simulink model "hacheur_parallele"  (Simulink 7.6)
settings: Solver=ode15s  StartTime=0.0  StopTime=20  RelTol=1e-3
InitFcn:
  | clc
StopFcn:
  | clc
  | close all, clc
  | load U_Umoy_charge.mat
  | plot(x(1,:),x(2,:),x(1,:),x(3,:))
  | xlabel('temps')
  | title('Tension charge et sa valeur moyenne')
  | grid
  | 
  | load I_Imoy_charge.mat
  | figure
  | plot(y(1,:),y(2,:),y(1,:),y(3,:))
  | xlabel('temps')
  | title('Courant charge et sa valeur moyenne')
  | grid
  | 
  | delete *.mat
libraries: fl_lib x15, powerlib x13, nesl_utility x6, elec_lib x4, powerlib_extras x2

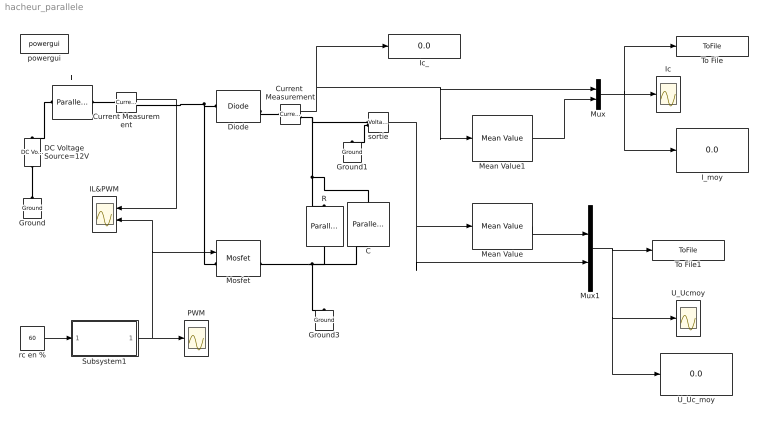
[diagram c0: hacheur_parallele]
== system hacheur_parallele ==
  C : powerlib/Elements/Parallel RLC Branch  DialogController=POWERSYS.PowerSysDialog  PhysicalDomain=powersysdomain  SubClassName=unknown  LeftPortType=p1  RightPortType=p1  LConnTagsString=a  RConnTagsString=__new0  BranchType=C  Resistance=1  Inductance=1e-3  SetiL0=off  InitialCurrent=0  Capacitance=100e-3  Setx0=off  InitialVoltage=0  Measurements=None
  Current Measurement : powerlib/Measurements/Current Measurement  DialogController=POWERSYS.PowerSysDialog  SystemSampleTime=-1  PhasorSimulation=off  OutputType=Complex  PSBequivalent=0
  Current  Measurement : powerlib/Measurements/Current Measurement  DialogController=POWERSYS.PowerSysDialog  SystemSampleTime=-1  PhasorSimulation=off  OutputType=Complex  PSBequivalent=0
  DC Voltage  Source=12V : powerlib/Electrical Sources/DC Voltage Source  DialogController=POWERSYS.PowerSysDialog  SystemSampleTime=-1  Amplitude=12  Measurements=None
  Diode : powerlib/Power Electronics/Diode  DialogController=POWERSYS.PowerSysDialog  SystemSampleTime=-1  Ron=0.001  Lon=0  Vf=0.8  IC=0  UseSnubber=off  Rs=500  Cs=250e-9  Measurements=on
  Ground : powerlib/Elements/Ground  DialogController=POWERSYS.PowerSysDialog  PhysicalDomain=powersysdomain  SubClassName=unknown  LeftPortType=p1  RightPortType=p1  LConnTagsString=a
  Ground1 : powerlib/Elements/Ground  DialogController=POWERSYS.PowerSysDialog  PhysicalDomain=powersysdomain  SubClassName=unknown  LeftPortType=p1  RightPortType=p1  LConnTagsString=a
  Ground3 : powerlib/Elements/Ground  DialogController=POWERSYS.PowerSysDialog  PhysicalDomain=powersysdomain  SubClassName=unknown  LeftPortType=p1  RightPortType=p1  LConnTagsString=a
  IL&PWM : Scope  NumInputPorts=2
  I_moy : Display
  Ic : Scope
  Ic_ : Display
  L : powerlib/Elements/Parallel RLC Branch  DialogController=POWERSYS.PowerSysDialog  PhysicalDomain=powersysdomain  SubClassName=unknown  LeftPortType=p1  RightPortType=p1  LConnTagsString=a  RConnTagsString=__new0  BranchType=L  Resistance=50  Inductance=1  SetiL0=off  InitialCurrent=0  Capacitance=25e-06  Setx0=off  InitialVoltage=0  Measurements=Branch voltage and current
  Mean Value : powerlib_extras/Measurements/Mean Value  DialogController=POWERSYS.PowerSysDialog  SystemSampleTime=-1  Period=10
  Mean Value1 : powerlib_extras/Measurements/Mean Value  DialogController=POWERSYS.PowerSysDialog  SystemSampleTime=-1  Period=10
  Mosfet : powerlib/Power Electronics/Mosfet  DialogController=POWERSYS.PowerSysDialog  SystemSampleTime=-1  Ron=0.1  Lon=0  Rd=0.01  Vfd=0  IC=0  Rs=1e5  Cs=inf  Measurements=on
  Mux : Mux  Inputs=2
  Mux1 : Mux  Inputs=2
  PWM : Scope
  R : powerlib/Elements/Parallel RLC Branch  DialogController=POWERSYS.PowerSysDialog  PhysicalDomain=powersysdomain  SubClassName=unknown  LeftPortType=p1  RightPortType=p1  LConnTagsString=a  RConnTagsString=__new0  BranchType=R  Resistance=10  Inductance=1.0  SetiL0=off  InitialCurrent=0  Capacitance=25e-06  Setx0=off  InitialVoltage=0  Measurements=Branch voltage and current
  Subsystem1 : Subsystem
  To File : ToFile  Filename=I_Imoy_charge  MatrixName=y
  To File1 : ToFile  Filename=U_Umoy_charge  MatrixName=x
  U_Uc_moy : Display
  U_Ucmoy : Scope
  powergui : powerlib/powergui  SystemSampleTime=-1  SimulationMode=Continuous  SampleTime=0  frequency=60  SPID=off  DisableSnubberDevices=off  DisableRonSwitches=off  DisableVfSwitches=off  SwTol=0  Interpol=off  frequencyindice=0  echomessages=off  HookPort=off  DisplayEquations=off  FunctionMessages=off  EnableUseOfTLC=off  x0status=blocks  RestoreLinks=warning  ResistiveCurrentMeasurement=off  Frange=[0:2:500]  Ylog=off  Xlog=on  ShowGrid=off  save=off  variable=ZData  ZoomFFT=on  StartTime=0.0  cycles=1  DisplayStyle=1  fundamental=60  FreqAxis=off  MaxFrequency=1000  frequencyindicesteady=1  RmsSteady=1  display=off  Ts=0  methode=off
  rc en % : Constant  Value=60
  sortie : powerlib/Measurements/Voltage Measurement  DialogController=POWERSYS.PowerSysDialog  SystemSampleTime=-1  PhasorSimulation=off  OutputType=Complex  PSBequivalent=0
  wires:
  rc en %/1 -> Subsystem1/1(rc (%))
  sortie/1 -> Mean Value/1, Mux1/2
  Current  Measurement/1 -> Ic_/1, Mean Value1/1, Mux/1
  Mean Value1/1 -> Mux/2
  Mux/1 -> Ic/1, To File/1, I_moy/1
  Subsystem1/1(PWM) -> PWM/1, Mosfet/1, IL&PWM/2
  Mean Value/1 -> Mux1/1
  Mux1/1 -> To File1/1, U_Uc_moy/1, U_Ucmoy/1
  Current Measurement/1 -> IL&PWM/1
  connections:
  DC Voltage  Source=12V/LConn1 -- Ground/LConn1
  Mosfet/RConn1 -- R/RConn1 -- Ground3/LConn1 -- C/LConn1
  sortie/LConn2 -- Ground1/LConn1
  Current  Measurement/RConn1 -- R/LConn1 -- C/RConn1 -- sortie/LConn1
  L/RConn1 -- DC Voltage  Source=12V/RConn1
  Mosfet/LConn1 -- Diode/LConn1 -- Current Measurement/RConn1
  Diode/RConn1 -- Current  Measurement/LConn1
  L/LConn1 -- Current Measurement/LConn1

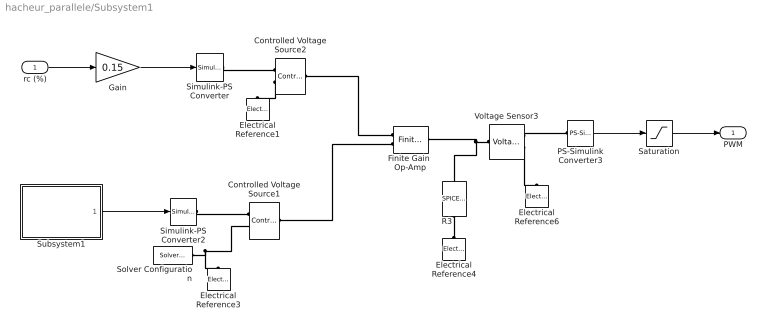
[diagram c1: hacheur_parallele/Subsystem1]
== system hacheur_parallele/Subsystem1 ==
  rc (%) : Inport
  Controlled Voltage Source1 : fl_lib/Electrical/Electrical Sources/Controlled Voltage Source  DialogController=NetworkEngine.DynNeDlgSource  SystemSampleTime=-1  i_Log=off  v_Log=off  LocalVarNames=|current|voltage|power  LocalVarDescs=|Current (A)|Voltage (V)|Power (W)  LocalVarLogging=[0 0 0]
  Controlled Voltage Source2 : fl_lib/Electrical/Electrical Sources/Controlled Voltage Source  DialogController=NetworkEngine.DynNeDlgSource  SystemSampleTime=-1  i_Log=off  v_Log=off  LocalVarNames=|current|voltage|power  LocalVarDescs=|Current (A)|Voltage (V)|Power (W)  LocalVarLogging=[0 0 0]
  Electrical Reference{1,3..4,6} (4 alike) : fl_lib/Electrical/Electrical Elements/Electrical Reference  DialogController=NetworkEngine.DynNeDlgSource  SystemSampleTime=-1  i_Log=off  LocalVarNames=|i  LocalVarDescs=|i  LocalVarLogging=[]
  Finite Gain  Op-Amp : elec_lib/Integrated Circuits/Finite Gain Op-Amp  DialogController=NetworkEngine.DynNeDlgSource  SystemSampleTime=-1  A=1000  Rin=1e+06 Ohm  Rout=100 Ohm  Vmin=-12 V  Vmax=12 V  LocalVarNames=|power  LocalVarDescs=|Dissipated power (W)  LocalVarLogging=0
  Gain : Gain  Gain=0.15
  PS-Simulink Converter3 : nesl_utility/PS-Simulink Converter  DialogController=NetworkEngine.DynNeUtilDlgSource  SystemSampleTime=-1  PhysicalDomain=network_engine_domain  LeftPortType=input  RightPortType=output  SubClassName=ps_output  Unit=1  AffineConversion=off
  R3 : elec_lib/Additional Components/SPICE-Compatible Components/Passive Devices/SPICE Resistor  DialogController=NetworkEngine.DynNeDlgSource  SystemSampleTime=-1  SCALE=1  R_param=1  R=10e3 Ohm  RSH=0 Ohm  LENGTH=1e-06 m  WIDTH=1e-06 m  NARROW=0 m  T_param=1  TC1=0 1/K  TC2=0 1/K^2  TOFFSET=0 K  TFIXED=300.15 K  TMEAS=300.15 K  LocalVarLogging=[]
  Saturation : Saturate  UpperLimit=1  LowerLimit=0
  Simulink-PS Converter : nesl_utility/Simulink-PS Converter  DialogController=NetworkEngine.DynNeUtilDlgSource  SystemSampleTime=-1  PhysicalDomain=network_engine_domain  LeftPortType=input  RightPortType=output  SubClassName=ps_input  Unit=1  AffineConversion=off  InputFilterTimeConstant=.001  UdotUserProvided=0
  Simulink-PS Converter2 : nesl_utility/Simulink-PS Converter  DialogController=NetworkEngine.DynNeUtilDlgSource  SystemSampleTime=-1  PhysicalDomain=network_engine_domain  LeftPortType=input  RightPortType=output  SubClassName=ps_input  Unit=1  AffineConversion=off  InputFilterTimeConstant=.001  UdotUserProvided=0
  Solver Configuration : nesl_utility/Solver Configuration  DialogController=NetworkEngine.DynNeUtilDlgSource  SystemSampleTime=-1  PhysicalDomain=network_engine_domain  LeftPortType=input  RightPortType=generic  SubClassName=solver  Accelerate=off  Profile=off  ResidualTolerance=1e-12  MaxNonlinIter=12  MaxModeIter=2  DoFixedCost=on  UseLocalSampling=off  DoDC=off  LinearAlgebra=Sparse  LocalSolverSampleTime=.001  LocalSolverChoice=NE_BACKWARD_EULER_ADVANCER  UseLocalSolver=off
  Subsystem1 : Subsystem
  Voltage Sensor3 : fl_lib/Electrical/Electrical Sensors/Voltage Sensor  DialogController=NetworkEngine.DynNeDlgSource  SystemSampleTime=-1  i1_Log=off  v1_Log=off  LocalVarNames=|i1|v1  LocalVarDescs=|i1|v1  LocalVarLogging=[]
  PWM : Outport
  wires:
  Gain/1 -> Simulink-PS Converter/1
  Saturation/1 -> PWM/1
  PS-Simulink Converter3/1 -> Saturation/1
  rc (%)/1 -> Gain/1
  Subsystem1/1(tri) -> Simulink-PS Converter2/1
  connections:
  Voltage Sensor3/RConn1 -- PS-Simulink Converter3/LConn1
  Voltage Sensor3/LConn1 -- R3/RConn1 -- Finite Gain  Op-Amp/RConn1
  Voltage Sensor3/RConn2 -- Electrical Reference6/LConn1
  Electrical Reference4/LConn1 -- R3/LConn1
  Controlled Voltage Source2/RConn2 -- Electrical Reference1/LConn1
  Simulink-PS Converter/RConn1 -- Controlled Voltage Source2/RConn1
  Finite Gain  Op-Amp/LConn1 -- Controlled Voltage Source2/LConn1
  Solver Configuration/RConn1 -- Electrical Reference3/LConn1 -- Controlled Voltage Source1/RConn2
  Simulink-PS Converter2/RConn1 -- Controlled Voltage Source1/RConn1
  Controlled Voltage Source1/LConn1 -- Finite Gain  Op-Amp/LConn2

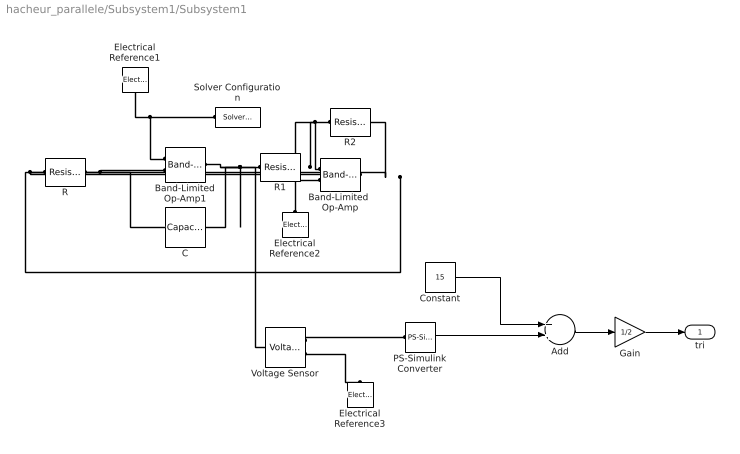
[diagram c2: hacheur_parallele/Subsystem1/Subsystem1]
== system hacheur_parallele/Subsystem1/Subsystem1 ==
  Add : Sum
  Band-Limited  Op-Amp : elec_lib/Integrated Circuits/Band-Limited Op-Amp  DialogController=NetworkEngine.DynNeDlgSource  SystemSampleTime=-1  A=1000  Rin=1e+06 Ohm  Rout=100 Ohm  Vmin=-15 V  Vmax=15 V  Vdotmax=1000 V/s  f=1e+05 Hz  V0=0 V  LocalVarNames=|power  LocalVarDescs=|Dissipated power (W)  LocalVarLogging=0
  Band-Limited Op-Amp1 : elec_lib/Integrated Circuits/Band-Limited Op-Amp  DialogController=NetworkEngine.DynNeDlgSource  SystemSampleTime=-1  A=1000  Rin=1e+06 Ohm  Rout=100 Ohm  Vmin=-15 V  Vmax=15 V  Vdotmax=1000 V/s  f=1e+05 Hz  V0=0 V  LocalVarNames=|power  LocalVarDescs=|Dissipated power (W)  LocalVarLogging=0
  C : fl_lib/Electrical/Electrical Elements/Capacitor  DialogController=NetworkEngine.DynNeDlgSource  SystemSampleTime=-1  c=0.5e-4 F  v0=0.1 V  r=1e-6 Ohm  g=0 1/Ohm  i_Log=off  v_Log=off  vc_Log=off  LocalVarNames=|current|voltage|power  LocalVarDescs=|Capacitor current (A)|Voltage across capacitor (V)|Power (W)  LocalVarLogging=[0 0 0]
  Constant : Constant  Value=15
  Electrical Reference1 : fl_lib/Electrical/Electrical Elements/Electrical Reference  DialogController=NetworkEngine.DynNeDlgSource  SystemSampleTime=-1  i_Log=off  LocalVarNames=|i  LocalVarDescs=|i  LocalVarLogging=[]
  Electrical Reference2 : fl_lib/Electrical/Electrical Elements/Electrical Reference  DialogController=NetworkEngine.DynNeDlgSource  SystemSampleTime=-1  i_Log=off  LocalVarNames=|i  LocalVarDescs=|i  LocalVarLogging=[]
  Electrical Reference3 : fl_lib/Electrical/Electrical Elements/Electrical Reference  DialogController=NetworkEngine.DynNeDlgSource  SystemSampleTime=-1  i_Log=off  LocalVarNames=|i  LocalVarDescs=|i  LocalVarLogging=[]
  Gain : Gain  Gain=1/2
  PS-Simulink Converter : nesl_utility/PS-Simulink Converter  DialogController=NetworkEngine.DynNeUtilDlgSource  SystemSampleTime=-1  PhysicalDomain=network_engine_domain  LeftPortType=input  RightPortType=output  SubClassName=ps_output  Unit=1  AffineConversion=off
  R : fl_lib/Electrical/Electrical Elements/Resistor  DialogController=NetworkEngine.DynNeDlgSource  SystemSampleTime=-1  R=1000 Ohm  i_Log=off  v_Log=off  LocalVarNames=|current|voltage|power  LocalVarDescs=|Resistor current (A)|Voltage across resistor (V)|Power (W)  LocalVarLogging=[0 0 0]
  R1 : fl_lib/Electrical/Electrical Elements/Resistor  DialogController=NetworkEngine.DynNeDlgSource  SystemSampleTime=-1  R=10e3 Ohm  i_Log=off  v_Log=off  LocalVarNames=|current|voltage|power  LocalVarDescs=|Resistor current (A)|Voltage across resistor (V)|Power (W)  LocalVarLogging=[0 0 0]
  R2 : fl_lib/Electrical/Electrical Elements/Resistor  DialogController=NetworkEngine.DynNeDlgSource  SystemSampleTime=-1  R=10e3 Ohm  i_Log=off  v_Log=off  LocalVarNames=|current|voltage|power  LocalVarDescs=|Resistor current (A)|Voltage across resistor (V)|Power (W)  LocalVarLogging=[0 0 0]
  Solver Configuration : nesl_utility/Solver Configuration  DialogController=NetworkEngine.DynNeUtilDlgSource  SystemSampleTime=-1  PhysicalDomain=network_engine_domain  LeftPortType=input  RightPortType=generic  SubClassName=solver  Accelerate=off  Profile=off  ResidualTolerance=1e-9  MaxNonlinIter=12  MaxModeIter=2  DoFixedCost=off  UseLocalSampling=off  DoDC=off  LinearAlgebra=Sparse  LocalSolverSampleTime=.001  LocalSolverChoice=NE_BACKWARD_EULER_ADVANCER  UseLocalSolver=off
  Voltage Sensor : fl_lib/Electrical/Electrical Sensors/Voltage Sensor  DialogController=NetworkEngine.DynNeDlgSource  SystemSampleTime=-1  i1_Log=off  v1_Log=off  LocalVarNames=|i1|v1  LocalVarDescs=|i1|v1  LocalVarLogging=[]
  tri : Outport
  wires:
  PS-Simulink Converter/1 -> Add/2
  Constant/1 -> Add/1
  Add/1 -> Gain/1
  Gain/1 -> tri/1
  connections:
  Voltage Sensor/RConn1 -- PS-Simulink Converter/LConn1
  Band-Limited Op-Amp1/RConn1 -- R1/LConn1 -- C/RConn1 -- Voltage Sensor/LConn1
  R/RConn1 -- C/LConn1 -- Band-Limited Op-Amp1/LConn2
  Solver Configuration/RConn1 -- Band-Limited Op-Amp1/LConn1 -- Electrical Reference1/LConn1
  R/LConn1 -- Band-Limited  Op-Amp/RConn1 -- R2/RConn1
  Electrical Reference2/LConn1 -- Band-Limited  Op-Amp/LConn2
  R2/LConn1 -- Band-Limited  Op-Amp/LConn1 -- R1/RConn1
  Voltage Sensor/RConn2 -- Electrical Reference3/LConn1
